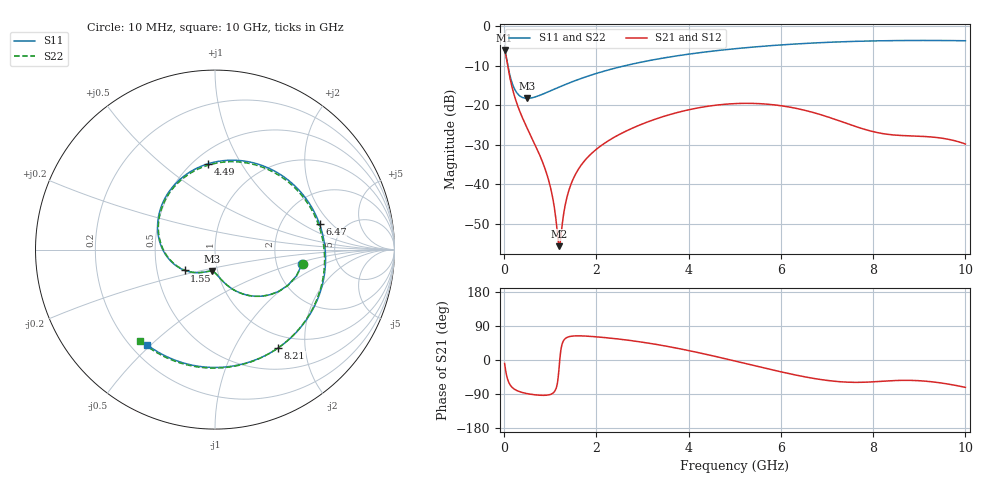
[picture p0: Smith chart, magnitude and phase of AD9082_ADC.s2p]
! Created Tue Jun 16 16:20:44 2020
# hz S ma R 50
! 2 Port Network Data from SP1.SP block
! freq  magS11  angS11  magS21  angS21  magS12  angS12  magS22  angS22
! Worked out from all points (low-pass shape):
!   1000 points, 10 MHz to 10 GHz, reference 50 ohm
!   highest |S21| = -6.17 dB at 10 MHz (marker M1); lowest = -55.7 dB at 1.2 GHz (marker M2)
!   |S21| within 3 dB of the highest: start of sweep to 64.16 MHz
!   lowest |S11| = -18.3 dB at 500 MHz (marker M3), VSWR 1.28, Z = 46.9 - j11.5 ohm
!   |S11| at or under -10 dB: 79.93 MHz to 2.635 GHz (2.555 GHz wide, 188 % of centre)
!   |S22| runs from -18.3 to -3.6 dB; largest |S21 - S12| = 0
!   S11 on the Smith chart (normalised r, x): 10 MHz: 2.80, -0.59; 1.55 GHz: 0.69, -0.17; 4.49 GHz: 0.59, +0.73; 6.47 GHz: 3.31, +1.45; 8.21 GHz: 0.80, -1.52; 10 GHz: 0.26, -0.49
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1e7  0.4927 -9.3  0.4916 -9.2  0.4916 -9.2  0.4941 -9.3
8e7  0.3161 -53.9  0.3068 -52.8  0.3068 -52.8  0.3172 -53.8
1.6e8  0.2002 -72.8  0.1792 -70.5  0.1792 -70.5  0.2011 -72.7
3e8  0.1373 -86.6  0.09567 -81.9  0.09567 -81.9  0.1377 -86.6
5e8  0.1217 -98.3  0.05099 -88.7  0.05099 -88.7  0.1215 -98.4
9.5e8  0.1468 -119.7  0.012 -92.4  0.012 -92.4  0.1461 -119.7
1.2e9  0.1697 -130.7  0.001646 -7.6  0.001646 -7.6  0.1688 -130.7
1.37e9  0.1865 -138.0  0.007147 60.0  0.007147 60.0  0.1854 -138.0
1.55e9  0.2049 -145.6  0.01347 63.7  0.01347 63.7  0.2035 -145.7
1.68e9  0.2183 -151.0  0.01775 63.6  0.01775 63.6  0.2168 -151.1
2.3e9  0.2824 -176.5  0.03664 57.7  0.03664 57.7  0.28 -176.7
3.34e9  0.3836 141.4  0.06834 40.3  0.06834 40.3  0.3792 140.8
4.49e9  0.4794 94.8  0.09808 11.9  0.09808 11.9  0.4737 93.6
5.01e9  0.5166 73.6  0.1045 -2.9  0.1045 -2.9  0.5108 72.0
5.7e9  0.5599 45.3  0.1028 -22.8  0.1028 -22.8  0.5548 43.1
6.47e9  0.5998 13.5  0.08728 -43.3  0.08728 -43.3  0.5962 10.8
6.67e9  0.6085 5.3  0.08155 -47.8  0.08155 -47.8  0.6055 2.4
7.41e9  0.6345 -25.0  0.05913 -58.3  0.05913 -58.3  0.6336 -28.4
8.21e9  0.6511 -57.3  0.04362 -56.0  0.04362 -56.0  0.6527 -61.0
8.34e9  0.6527 -62.4  0.04255 -55.0  0.04255 -55.0  0.6547 -66.2
9.14e9  0.6566 -93.5  0.04002 -55.9  0.04002 -55.9  0.6608 -97.3
1e10  0.6512 -125.6  0.03222 -72.2  0.03222 -72.2  0.6571 -129.4
